[IBIS Ver]   3.2
[File name]   sprm135a.ibs
[File Rev]   1.1
[Date]   Tue Mar 4 14:22:13 US/Central 2003
[Source]   IBIS Model Generated from PACED 4.51D
|   Technology type SR40
[Disclaimer]   Please be aware that in the absence of a written agreement
|   Texas Instruments(TI) assumes no liability for:
|   (1) The accuracy of the IBIS models provided to your company
|   (2) The proper functioning of these Models in your design
|   or for any resulting applications;or
|   property rights resulting from your use of these models.
|   TI provides IBIS Models as a service to our customers and
|   therefore reserves the right to limit distribution of the
|   Models.
[Copyright]   Property of Texas Instruments Incorporated.
|   Unauthorised reproduction and/or distribution is strictly.
|   prohibited.
|   This product is protected under copyright law and trade
|   secret law as an unpublished work.
|   Created 1999,(C) Copyright 1999-2001,
|   Texas Instruments Incorporated., All Rights Reserved.
[Notes]
|   File Rev 1.0:   Original
|   File Rev 1.1:   Corrected EMIF address pin names.
|   Corrected EMIF clock pin names.
|   Removed PLLSENSE pin, this pin is NC pin.
[Component]   TMS320VC5502_GZZ   | 176 pin (not including 25 thermal balls)
[Manufacturer]   Texas Instruments
[Package]
| Variable   Typ   Min   Max
R_pkg   0.2117   0.1771   0.2537
L_pkg   3.208e-09   2.166e-09   5.003e-09
C_pkg   2.837e-13   1.526e-13   4.605e-13
[Pin]  signal_name   model_name   R_pin   L_pin   C_pin
A2   GPIO7   idi041_ouk831   0.2470   4.847e-09   4.187e-13
A3   GND   NC   0.2409   4.373e-09   4.461e-13
A4   POWER   NC   0.2349   4.136e-09   3.854e-13
A5   POWER   NC   0.2286   3.864e-09   3.185e-13
A6   POWER   NC   0.2194   3.624e-09   3.012e-13
A7   TMS   idi041_ps1001   0.2122   3.446e-09   3.159e-13
A8   GND   NC   0.2064   3.392e-09   3.274e-13
A9   GND   NC   0.2079   3.477e-09   2.861e-13
A10   D3   ups312_ouk831   0.2145   3.522e-09   3.461e-13
A11   POWER   NC   0.2118   3.420e-09   3.682e-13
A12   GND   NC   0.2212   3.596e-09   2.876e-13
A13   POWER   NC   0.2301   3.914e-09   3.427e-13
A14   D11   ups312_ouk831   0.2336   4.179e-09   3.888e-13
A15   D14   ups312_ouk831   0.2425   4.458e-09   4.602e-13
A16   D16   ups312_ouk831   0.2499   4.917e-09   4.236e-13
B1   GPIO6   idi041_ouk831   0.2533   5.001e-09   4.369e-13
B3   HD0   ups312_ouk831   0.2249   3.809e-09   4.270e-13
B4   HD2   ups312_ouk831   0.2197   3.501e-09   3.361e-13
B5   HD4   ups312_ouk831   0.2094   3.143e-09   2.793e-13
B6   HD6   ups312_ouk831   0.2070   3.066e-09   2.699e-13
B7   NRESET   idg091   0.1984   2.845e-09   2.797e-13
B8   TDI   idi041_ps1001   0.1919   2.812e-09   2.652e-13
B9   TDO   ouk831   0.1918   2.812e-09   2.673e-13
B10   D0   ups312_ouk831   0.1931   2.793e-09   2.395e-13
B11   D4   ups312_ouk831   0.1991   2.909e-09   2.738e-13
B12   D7   ups312_ouk831   0.2063   3.011e-09   2.600e-13
B13   D9   ups312_ouk831   0.2132   3.254e-09   3.104e-13
B14   D12   ups312_ouk831   0.2165   3.535e-09   3.588e-13
B15   D15   ups312_ouk831   0.2270   3.870e-09   4.340e-13
B17   D17   ups312_ouk831   0.2489   4.855e-09   4.175e-13
C1   GPIO2   idi041_ouk831   0.2459   4.428e-09   4.424e-13
C2   GPIO4   idi041_ouk831   0.2290   3.854e-09   4.316e-13
C4   HD1   ups312_ouk831   0.2032   2.863e-09   2.491e-13
C5   HD3   ups312_ouk831   0.1948   2.553e-09   2.132e-13
C6   HD5   ups312_ouk831   0.1925   2.401e-09   1.856e-13
C7   HPIENA   idg091   0.1876   2.270e-09   1.807e-13
C8   TCK   idi091_ps1001   0.1810   2.194e-09   1.607e-13
C9   EMU0   idi041_ouk831_ps1001 0.1787   2.166e-09   1.665e-13
C10   D1   ups312_ouk831   0.1817   2.201e-09   1.825e-13
C11   D5   ups312_ouk831   0.1873   2.267e-09   1.725e-13
C12   D8   ups312_ouk831   0.1916   2.381e-09   1.831e-13
C13   D10   ups312_ouk831   0.1979   2.674e-09   2.220e-13
C14   D13   ups312_ouk831   0.2032   2.938e-09   2.829e-13
C16   D18   ups312_ouk831   0.2267   3.827e-09   4.237e-13
C17   GND   NC   0.2426   4.400e-09   4.436e-13
D1   TIM1   idi041_ouk831   0.2376   4.167e-09   3.799e-13
D2   GPIO0   idi041_ouk831   0.2215   3.530e-09   3.265e-13
D3   GPIO1   idi041_ouk831   0.2061   2.902e-09   2.538e-13
D7   HD7   ups312_ouk831   0.1880   2.352e-09   1.543e-13
D8   TRSTN   idg091_pe1001   0.1785   2.234e-09   1.630e-13
D9   EMU1   idi041_ouk831_ps1001 0.1771   2.221e-09   1.566e-13
D10   D2   ups312_ouk831   0.1814   2.268e-09   1.619e-13
D11   D6   ups312_ouk831   0.1877   2.348e-09   1.543e-13
D15   D19   ups312_ouk831   0.2070   2.905e-09   2.488e-13
D16   D20   ups312_ouk831   0.2233   3.548e-09   3.391e-13
D17   D21   ups312_ouk831   0.2384   4.179e-09   3.868e-13
E1   POWER   NC   0.2335   3.961e-09   3.542e-13
E2   NINT0   idg091   0.2166   3.226e-09   2.945e-13
E3   TIM0   idi041_ouk831   0.2013   2.683e-09   2.259e-13
E15   D22   ups312_ouk831   0.2011   2.624e-09   2.155e-13
E16   D23   ups312_ouk831   0.2164   3.218e-09   2.942e-13
E17   POWER   NC   0.2344   3.905e-09   3.310e-13
F1   POWER   NC   0.2311   3.709e-09   2.925e-13
F2   NINT2   idg091   0.2157   3.121e-09   2.659e-13
F3   NINT1   idg091   0.2004   2.484e-09   1.868e-13
F15   D24   ups312_ouk831   0.2010   2.501e-09   1.926e-13
F16   D25   ups312_ouk831   0.2172   3.175e-09   2.640e-13
F17   POWER   NC   0.2309   3.739e-09   3.005e-13
G1   GND   NC   0.2240   3.563e-09   3.740e-13
G2   NIACK   ouk831   0.2109   3.046e-09   2.787e-13
G3   NNMI   idg091_ouk831_ps1001 0.1986   2.399e-09   1.756e-13
G4   NINT3   idg091   0.1983   2.472e-09   1.590e-13
G14   D26   ups312_ouk831   0.2004   2.499e-09   1.567e-13
G15   D27   ups312_ouk831   0.2005   2.422e-09   1.879e-13
G16   D28   ups312_ouk831   0.2116   3.000e-09   2.848e-13
G17   GND   NC   0.2257   3.607e-09   3.210e-13
H1   CLKR0   idg091_ouk831   0.2259   3.656e-09   3.500e-13
H2   CLKX0   idg091_ouk831   0.2065   2.950e-09   2.451e-13
H3   FSR0   idi041_ouk831   0.1946   2.351e-09   1.877e-13
H4   DR0   idg041   0.1935   2.410e-09   1.673e-13
H14   D30   ups312_ouk831   0.1938   2.413e-09   1.687e-13
H15   D29   ups312_ouk831   0.1962   2.373e-09   1.651e-13
H16   D31   ups312_ouk831   0.2072   2.990e-09   2.716e-13
H17   POWER   NC   0.2218   3.570e-09   3.304e-13
J1   POWER   NC   0.2223   3.646e-09   2.921e-13
J2   CLKR1   idg091_ouk831   0.2077   2.999e-09   2.738e-13
J3   FSX0   idi041_ouk831   0.1943   2.349e-09   1.731e-13
J4   DX0   ouk831   0.1923   2.399e-09   1.605e-13
J14   A4   ups312_ouk831   0.1923   2.399e-09   1.612e-13
J15   A3   ups312_ouk831   0.1940   2.346e-09   1.726e-13
J16   A2   ups312_ouk831   0.2071   2.992e-09   2.727e-13
J17   GND   NC   0.2224   3.648e-09   2.909e-13
K1   DR1   idg041   0.2226   3.587e-09   3.338e-13
K2   FSR1   idi041_ouk831   0.2075   2.994e-09   2.704e-13
K3   CLKX1   idg091_ouk831   0.1967   2.379e-09   1.650e-13
K4   DX1   ouk831   0.1942   2.418e-09   1.685e-13
K14   A7   ups312_ouk831   0.1945   2.422e-09   1.678e-13
K15   A6   ups312_ouk831   0.1953   2.361e-09   1.874e-13
K16   A5   ups312_ouk831   0.2071   2.957e-09   2.457e-13
K17   POWER   NC   0.2281   3.652e-09   3.415e-13
L1   GND   NC   0.2266   3.613e-09   3.205e-13
L2   FSX1   idi041_ouk831   0.2126   3.011e-09   2.842e-13
L3   DR2   idg041   0.2016   2.434e-09   1.852e-13
L4   DX2   ouk831   0.2016   2.512e-09   1.579e-13
L14   A11   ups312_ouk831   0.2001   2.495e-09   1.590e-13
L15   A10   ups312_ouk831   0.2003   2.419e-09   1.725e-13
L16   A9   ups312_ouk831   0.2124   3.068e-09   2.792e-13
L17   A8   ups312_ouk831   0.2254   3.580e-09   3.736e-13
M1   POWER   NC   0.2320   3.743e-09   3.031e-13
M2   SP3   idi041_ouk831   0.2186   3.187e-09   2.709e-13
M3   SP2   idi041_ouk831   0.2026   2.519e-09   1.939e-13
M15   A13   ups312_ouk831   0.2008   2.497e-09   2.038e-13
M16   A12   ups312_ouk831   0.2157   3.079e-09   2.682e-13
M17   POWER   NC   0.2321   3.710e-09   3.016e-13
N1   POWER   NC   0.2362   3.926e-09   3.318e-13
N2   SP1   idg091_ouk831   0.2183   3.241e-09   2.946e-13
N3   SP0   idg091_ouk831   0.2032   2.649e-09   2.171e-13
N15   A15   ups312_ouk831   0.2008   2.658e-09   2.182e-13
N16   A14   ups312_ouk831   0.2172   3.235e-09   2.954e-13
N17   GND   NC   0.2342   3.865e-09   3.359e-13
P1   GND   NC   0.2407   4.206e-09   3.880e-13
P2   SCL   idi091_uos205   0.2258   3.578e-09   3.401e-13
P3   SDA   idi091_uos205   0.2097   2.936e-09   2.481e-13
P7   C15   ups312_ouk831   0.1874   2.344e-09   1.544e-13
P8   X1   NC   0.1800   2.252e-09   1.622e-13
P9   C13   ups312_ouk831   0.1771   2.221e-09   1.554e-13
P10   C8   ups312_ouk831   0.1789   2.238e-09   1.635e-13
P11   ECLKOUT1   ouk831   0.1892   2.367e-09   1.526e-13
P15   A17   ups312_ouk831   0.2036   2.903e-09   2.654e-13
P16   A16   ups312_ouk831   0.2220   3.532e-09   3.320e-13
P17   POWER   NC   0.2381   4.172e-09   3.792e-13
R1   HC1   idg091_ouk831_pe1001 0.2414   4.389e-09   4.425e-13
R2   HC0   idg091_ouk831_ps1001 0.2256   3.817e-09   4.214e-13
R4   HRNW   idi041_ouk831_ps1001 0.2030   2.940e-09   2.852e-13
R5   NHDS1   idg091_ouk831_ps1001 0.1974   2.669e-09   2.222e-13
R6   CLKOUT   oukb31   0.1911   2.375e-09   1.829e-13
R7   C14   idi041_ouk831_ps1001 0.1870   2.263e-09   1.715e-13
R8   X2CLKIN   NC   0.1805   2.187e-09   1.827e-13
R9   C12   ups312_ouk831   0.1787   2.166e-09   1.667e-13
R10   C7   ups312_ouk831   0.1815   2.200e-09   1.611e-13
R11   ECLKOUT2   ouk831   0.1887   2.283e-09   1.812e-13
R12   C5   ups312_ouk831   0.1893   2.354e-09   1.827e-13
R13   C3   idi041_ouk831_ps1001 0.1963   2.692e-09   2.274e-13
R14   C1   ups312_ouk831   0.2035   2.944e-09   2.866e-13
R16   A18   ups312_ouk831   0.2294   3.857e-09   4.304e-13
R17   GND   NC   0.2443   4.414e-09   4.399e-13
T1   NHCS   idg091_ouk831_ps1001 0.2479   4.849e-09   4.164e-13
T3   HCNTL0   idi041_ouk831_ps1001 0.2269   3.869e-09   4.337e-13
T4   NHDS2   idg091_ouk831_ps1001 0.2172   3.536e-09   3.613e-13
T5   HRDY   idi041_ouk831_ps1001 0.2127   3.248e-09   3.103e-13
T6   XF   ouk831   0.2061   3.008e-09   2.603e-13
T7   NHINT   idi041_ouk831_ps1001 0.1988   2.905e-09   2.742e-13
T8   EMIFCLKS   idg091   0.1921   2.781e-09   2.395e-13
T9   C11   ups312_ouk831   0.1919   2.814e-09   2.676e-13
T10   C9   ups312_ouk831   0.1922   2.838e-09   2.695e-13
T11   ECLKIN   idg091   0.2004   2.891e-09   2.885e-13
T12   C6   ups312_ouk831   0.2041   2.971e-09   2.599e-13
T13   C4   ups312_ouk831   0.2117   3.241e-09   3.085e-13
T14   C2   ups312_ouk831   0.2177   3.542e-09   3.594e-13
T15   A21   ups312_ouk831   0.2275   3.876e-09   4.330e-13
T17   A19   ups312_ouk831   0.2537   5.003e-09   4.373e-13
U2   HCNTL1   idi041_ouk831_ps1001 0.2499   4.917e-09   4.234e-13
U3   GND   NC   0.2424   4.455e-09   4.605e-13
U4   POWER   NC   0.2333   4.175e-09   3.891e-13
U5   POWER   NC   0.2296   3.908e-09   3.430e-13
U6   GND   NC   0.2209   3.593e-09   2.866e-13
U7   POWER   NC   0.2115   3.416e-09   3.693e-13
U8   NC01   NC   0.2129   3.504e-09   3.460e-13
U9   GND   NC   0.2073   3.470e-09   2.859e-13
U10   C10   ups312_ouk831   0.2066   3.396e-09   3.268e-13
U11   GND   NC   0.2130   3.456e-09   3.169e-13
U12   POWER   NC   0.2209   3.617e-09   2.858e-13
U13   POWER   NC   0.2277   3.915e-09   3.511e-13
U14   GND   NC   0.2337   4.201e-09   3.906e-13
U15   C0   ups312_ouk831   0.2429   4.472e-09   4.590e-13
U16   A20   ups312_ouk831   0.2495   4.914e-09   4.237e-13
| Models and submodels in the file (14): idg041 (Input), idg091 (Input), ouk831 (3-state), oukb31 (3-state), idg091_ouk831 (I/O), idg091_ouk831_ps1001 (I/O), idg091_pe1001 (Input), idi041_ouk831 (I/O), idi041_ouk831_ps1001 (I/O), idi041_ps1001 (Input), idi091_ps1001 (Input), idi091_uos205 (I/O_open_drain), ups312_ouk831 (I/O), idg091_ouk831_pe1001 (I/O)
